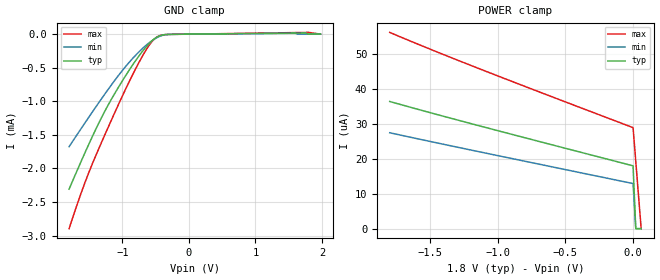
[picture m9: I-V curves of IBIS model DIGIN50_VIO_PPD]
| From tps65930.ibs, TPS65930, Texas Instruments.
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|   Model DIGIN50_VIO_PPD
[Model]   DIGIN50_VIO_PPD
Model_type   Input
Polarity   Non-Inverting
Vinl =   0.6930V
Vinh =   1.0530V
C_comp   56.6670fF   54.6940fF   53.5477fF
[Temperature Range]   25.0000   0.1250k   -40.0000
[Pullup Reference]   1.8000V   1.6200V   1.9800V
[Pulldown Reference]   0.000V   0.000V   0.000V
[POWER Clamp Reference]   1.8000V   1.6200V   1.9800V
[GND Clamp Reference]   0.000V   0.000V   0.000V
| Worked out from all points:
|   GND clamp passes 1 mA (typ) near -1.18 V on its own axis
[GND_clamp]
| voltage   I(typ)   I(min)   I(max)
-1.8V     -2.308mA   -1.676mA   -2.897mA
-1.52V    -1.675mA   -1.261mA   -2.102mA
-1.32V    -1.257mA   -972.1uA   -1.628mA
-1.16V    -962uA     -750.3uA   -1.271mA
-920mV    -571.5uA   -446.3uA   -755.6uA
-720mV    -285.5uA   -235uA     -366.9uA
-600mV    -143.5uA   -131.1uA   -169.8uA
-480mV    -43.64uA   -51.61uA   -42.38uA
-240mV    -2.436uA   -2.272uA   -3.503uA
1.76V     17.57uA    0A         25.67uA
1.8V      0A         0A         26.26uA
1.98V     0A         0A         0A
[POWER_clamp]
| voltage   I(typ)   I(min)   I(max)
-1.8V     36.38uA    27.44uA    56.14uA
-1.14V    29.45uA    22.01uA    45.79uA
0V        17.97uA    12.9uA     28.9uA
20mV      0A         0A         19.26uA
60mV      0A         0A         0A
